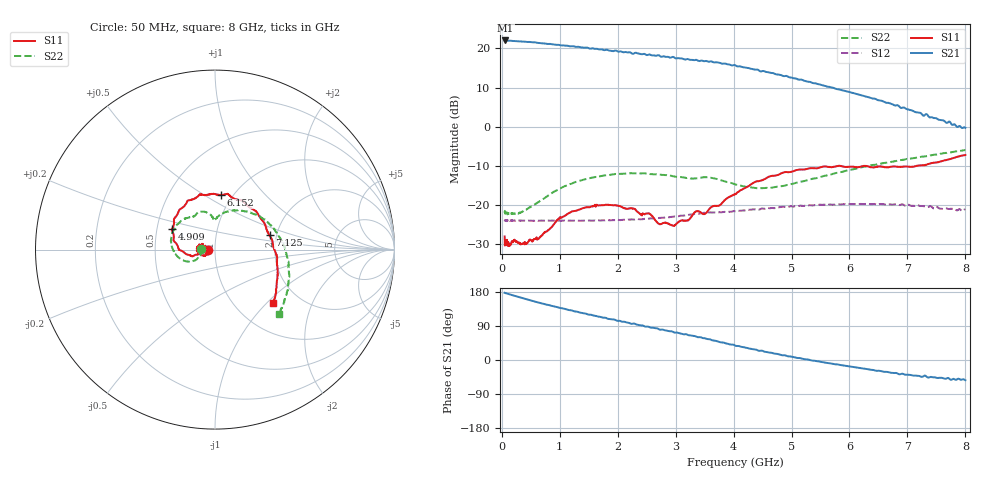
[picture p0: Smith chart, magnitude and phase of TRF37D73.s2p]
! Network Analyzer HP8720D.06.14 Serial No. US36140363
! Hewlett-Packard
! 27 May 2014  22:00:35
! Frequency  S11  S21  S12  S22
# HZ  S  DB R 50
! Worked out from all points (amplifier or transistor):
!   1601 points, 50 MHz to 8 GHz, reference 50 ohm
!   highest |S21| = 22.0 dB at 64.91 MHz (marker M1)
!   |S21| within 3 dB of that: start of sweep to 2.098 GHz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
!   unconditionally stable (mu >= 1): start of sweep to end of sweep
!   at 1.372 GHz: K = 1.06, MAG = 20.6 dB, |S12| = -23.9 dB
!   at 4.025 GHz: K = 1.20, MAG = 16.0 dB, |S12| = -21.6 dB
!   at 8 GHz: K = 3.41, MAG = 2.2 dB, |S12| = -21.2 dB
!   S11 on the Smith chart (normalised r, x): 50 MHz: 0.92, -0.00; 4.909 GHz: 0.60, +0.15; 6.152 GHz: 0.88, +0.59; 7.125 GHz: 1.84, +0.33; 8 GHz: 1.47, -1.08
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5e7  -27.98 -178.9  22.01 177.3  -24.11 1.0  -21.92 179.0
6.490625e7  -29.64 179.3  22.03 176.6  -23.90 1.4  -21.76 180.0
3.630312e8  -29.88 -172.1  21.75 163.1  -23.91 2.1  -21.61 -162.4
5.766875e8  -28.53 -161.5  21.54 153.9  -23.95 3.8  -19.73 -154.6
7.2575e8  -27.12 -147.3  21.29 148.0  -23.91 4.9  -18.32 -151.4
1.118281e9  -22.37 -154.6  20.71 133.6  -23.96 7.5  -14.96 -159.0
1.376656e9  -20.89 -165.4  20.26 124.5  -23.92 9.8  -13.64 -167.9
1.615156e9  -20.13 -175.5  19.89 116.8  -23.89 12.0  -12.80 -177.0
1.977875e9  -20.07 171.2  19.42 104.2  -23.71 15.2  -12.01 168.4
2.261094e9  -20.87 162.2  18.61 95.8  -23.61 17.4  -11.87 156.9
2.335625e9  -21.61 161.9  18.78 93.1  -23.51 18.4  -11.88 154.2
2.703312e9  -24.67 160.8  18.27 81.9  -23.25 21.8  -12.11 139.9
3.105781e9  -23.86 -177.0  17.44 69.2  -22.64 24.7  -12.83 126.9
3.632469e9  -20.30 -170.6  16.62 52.1  -21.87 24.6  -13.06 107.9
4.025e9  -17.19 -165.5  15.74 38.1  -21.55 25.7  -14.67 95.1
4.407594e9  -13.87 179.4  14.62 26.2  -21.05 25.6  -15.65 91.4
4.909438e9  -11.52 154.7  13.00 11.3  -20.41 24.0  -14.86 86.0
5.351656e9  -10.53 131.4  11.26 -1.5  -20.07 21.7  -13.29 74.5
6.151625e9  -10.30 83.6  8.28 -20.7  -19.69 17.0  -10.51 40.9
6.678312e9  -10.30 48.5  6.10 -32.3  -19.77 13.0  -9.06 16.8
7.1255e9  -10.05 14.8  3.82 -41.4  -20.15 10.0  -7.94 -4.5
8e9  -7.19 -42.8  -0.24 -53.4  -21.18 4.1  -5.91 -45.1
